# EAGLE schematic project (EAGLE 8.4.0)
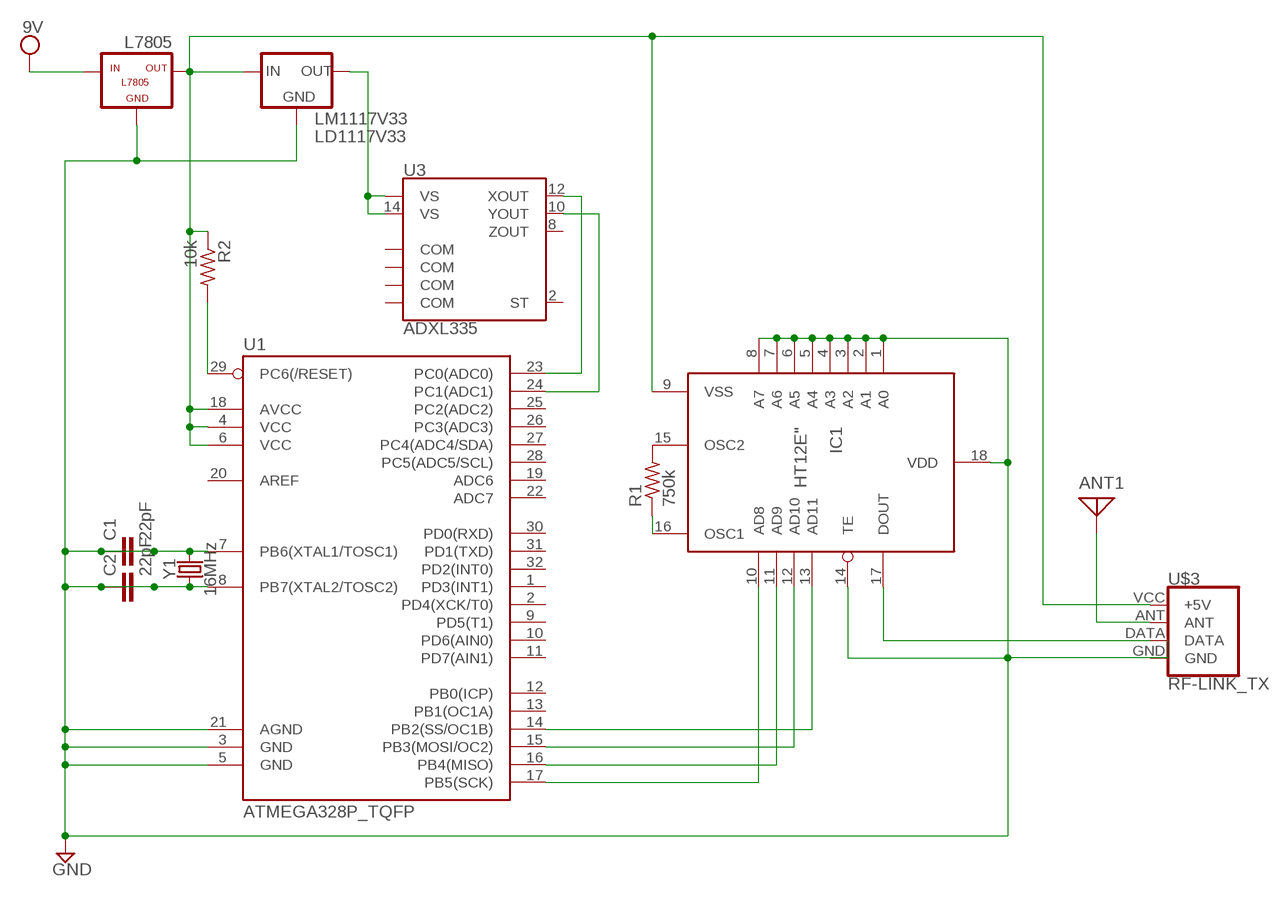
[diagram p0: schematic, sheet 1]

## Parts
ANT1  ANTENNA  [PAD-01]
C1  22pF  C-EUHPC0201  [HPC0201]
C2  22pF  C-EUHPC0201  [HPC0201]
IC1  HT12E"  [18-DIP-A]
L7805  5V  L7805  [78XXL]
LM1117V33  LD1117V33  [LD1117V33]
R1  750k  R-US_R0201  [R0201]
R2  10k  R-US_R0201  [R0201]
U1  ATMEGA328P_TQFP  [TQFP32-08]
U3  ADXL335  [LFCSP-16-4X4]
U$3  RF-LINK_TX  [RF-LINK_TX]
Y1  16MHz  CRYSTALPTH-HC49US  [HC49US]

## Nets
+5V: IC1.9(VSS) L7805.IN L7805.OUT LM1117V33.IN R2.1 U1.4(VCC) U1.6(VCC) U1.18(AVCC) U$3.VCC(+5V) ; supply symbol labelled 9V
GND: C1.1 C1.2 C2.1 C2.2 IC1.1(A0) IC1.2(A1) IC1.3(A2) IC1.4(A3) IC1.5(A4) IC1.6(A5) IC1.7(A6) IC1.8(A7) IC1.14(TE) IC1.18(VDD) L7805.GND LM1117V33.GND U1.3(GND) U1.5(GND) U1.7(PB6(XTAL1/TOSC1)) U1.8(PB7(XTAL2/TOSC2)) U1.21(AGND) Y1.1 Y1.2
N$1: IC1.16(OSC1) R1.1
N$2: IC1.13(AD11) U1.14(PB2(SS/OC1B))
N$3: IC1.12(AD10) U1.15(PB3(MOSI/OC2))
N$4: LM1117V33.OUT U3.14(VS) U3.15(VS)
N$5: IC1.17(DOUT) U$3.DATA
N$6: U1.23(PC0(ADC0)) U3.12(XOUT)
N$7: IC1.11(AD9) U1.16(PB4(MISO))
N$8: IC1.10(AD8) U1.17(PB5(SCK))
N$9: R2.2 U1.29(PC6(/RESET))
N$10: IC1.15(OSC2) R1.2
N$12: ANT1.1 U$3.ANT
N$13: U1.24(PC1(ADC1)) U3.10(YOUT)
Unconnected: U1.1(PD3(INT1)) U1.2(PD4(XCK/T0)) U1.9(PD5(T1)) U1.10(PD6(AIN0)) U1.11(PD7(AIN1)) U1.12(PB0(ICP)) U1.13(PB1(OC1A)) U1.19(ADC6) U1.20(AREF) U1.22(ADC7) U1.25(PC2(ADC2)) U1.26(PC3(ADC3)) U1.27(PC4(ADC4/SDA)) U1.28(PC5(ADC5/SCL)) U1.30(PD0(RXD)) U1.31(PD1(TXD)) U1.32(PD2(INT0)) U3.2(ST) U3.3(COM) U3.5(COM) U3.6(COM) U3.7(COM) U3.8(ZOUT)

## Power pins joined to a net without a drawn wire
GND: U$3.GND

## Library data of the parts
ANT1 = discrete:ANTENNA: Antenna
C1 C2 = resistor:C-EU: CAPACITOR, European symbol
IC1 = holtek:HT12E: transmitter = encoder ic
L7805 = l7805:L7805: VOLTAGE REGULATOR
LM1117V33 = lm1117v33:LD1117V33
R1 R2 = resistor:R-US_: RESISTOR, American symbol
U1 = SparkFun-IC-Microcontroller:ATMEGA328P_TQFP: Popular 328P in QFP Storefront component: ATmega328 - TQFP (COM-13448) Datasheet SparkFun Products SparkFun RedBoard - Programmed with Arduino (DEV-12757) Arduino Pro Mini 328 - 5V/16MHz (DEV-11113) Arduino Pro Mini 328 - 3.3V/8MHz (DEV-11114) SparkFun OpenLog (DEV-13712) SparkFun MicroView - OLED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; PROD_ID: IC-09069
U3 = SparkFun-Sensors:ADXL335: Analog Devices ADXL335 3-Axis Analog Accelerometer The ADXL335 is a small, thin, low power, complete 3-axis accelerometer with signal conditioned voltage outputs. The product measures acceleration with a minimum full-scale range of ±3 g. It can measure the static acceleration of gravity in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; PROD_ID: IC-08942; SF_ID: COM-09265
U$3 = SparkFun-RF:RF-LINK_TX: RF Link Transmitter (434 MHz, 315 MHz) These wireless transmitters work with equivalent receivers. They can easily fit into a breadboard and work well with microcontrollers to create a very simple wireless data link. Since these are only transmitters, they will only work communicating data one-way,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; SF_ID: WRL-10534
Y1 = SparkFun-Clocks:CRYSTAL: Crystals (Generic)

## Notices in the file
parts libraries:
SparkFun-IC-Microcontroller: Licensing: Creative Commons ShareAlike 4.0 International - https://creativecommons.org/licenses/by-sa/4.0
